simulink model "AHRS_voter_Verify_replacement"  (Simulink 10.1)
settings: Solver=FixedStepDiscrete  StartTime=0.0  StopTime=10.0  RelTol=1e-3
undefined symbols (not defined in the file or in its folder): sldvsubsys
libraries: simulink x2, sldvlib x1

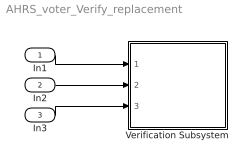
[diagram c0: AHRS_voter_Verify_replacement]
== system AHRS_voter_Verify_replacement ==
  In1 : Inport  OutDataTypeStr=Bus: AHRS_Bus
  In2 : Inport  Port=2  OutDataTypeStr=Bus: AHRS_Bus
  In3 : Inport  Port=3  OutDataTypeStr=Bus: AHRS_Bus
  Verification Subsystem : Subsystem  Tag=VerificationSubsystem  DisableCoverage=on  LoadFcn=sldvsubsys('check')  TreatAsAtomicUnit=on  SimViewingDevice=on
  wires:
  In1/1 -> Verification Subsystem/1(In1)
  In2/1 -> Verification Subsystem/2(In2)
  In3/1 -> Verification Subsystem/3(In3)

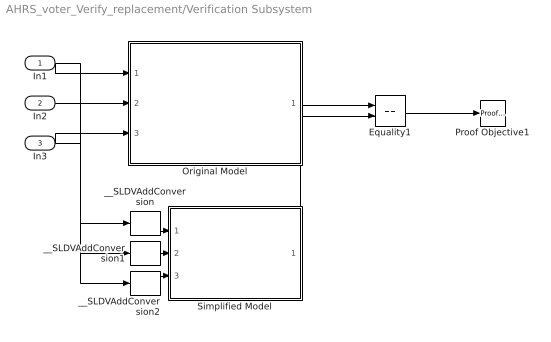
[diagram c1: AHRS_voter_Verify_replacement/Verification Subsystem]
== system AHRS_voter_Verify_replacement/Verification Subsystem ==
  In1 : Inport  OutDataTypeStr=Bus: AHRS_Bus
  In2 : Inport  Port=2  OutDataTypeStr=Bus: AHRS_Bus
  In3 : Inport  Port=3  OutDataTypeStr=Bus: AHRS_Bus
  Equality1 : RelationalOperator  Operator===  OutDataTypeStr=boolean  RndMeth=Simplest
  Original Model : Subsystem  TreatAsAtomicUnit=on
  Proof Objective1 : sldvlib/Objectives and Constraints/Proof Objective  enabled=on  customAVTBlockType=Proof Objective  intervals=true  dispValues=on  outEnabled=off  enableStopSim=off
  Simplified Model : Subsystem  TreatAsAtomicUnit=on
  __SLDVAddConversion : SignalConversion  ConversionOutput=Nonvirtual bus  OutDataTypeStr=Bus:AHRS_Bus  OverrideOpt=off
  __SLDVAddConversion1 : SignalConversion  ConversionOutput=Nonvirtual bus  OutDataTypeStr=Bus:AHRS_Bus  OverrideOpt=off
  __SLDVAddConversion2 : SignalConversion  ConversionOutput=Nonvirtual bus  OutDataTypeStr=Bus:AHRS_Bus  OverrideOpt=off
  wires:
  In1/1 -> Original Model/1(AHRS1), __SLDVAddConversion/1
  In2/1 -> Original Model/2(AHRS2), __SLDVAddConversion1/1
  In3/1 -> Original Model/3(AHRS3), __SLDVAddConversion2/1
  Original Model/1(voted_fb) -> Equality1/1
  Simplified Model/1(voted_fb) -> Equality1/2
  Equality1/1 -> Proof Objective1/1
  __SLDVAddConversion/1 -> Simplified Model/1(AHRS1)
  __SLDVAddConversion1/1 -> Simplified Model/2(AHRS2)
  __SLDVAddConversion2/1 -> Simplified Model/3(AHRS3)

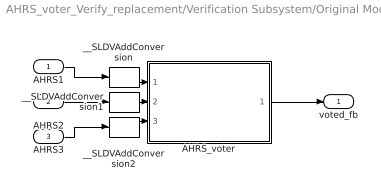
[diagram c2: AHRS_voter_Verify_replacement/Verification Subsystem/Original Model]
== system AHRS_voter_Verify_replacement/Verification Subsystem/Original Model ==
  AHRS1 : Inport  OutDataTypeStr=Bus: AHRS_Bus  SampleTime=[0.01,0]
  AHRS2 : Inport  Port=2  OutDataTypeStr=Bus: AHRS_Bus  SampleTime=[0.01,0]
  AHRS3 : Inport  Port=3  OutDataTypeStr=Bus: AHRS_Bus  SampleTime=[0.01,0]
  AHRS_voter : Subsystem  TreatAsAtomicUnit=on
  __SLDVAddConversion : SignalConversion  ConversionOutput=Nonvirtual bus  OutDataTypeStr=Bus:AHRS_Bus  OverrideOpt=off
  __SLDVAddConversion1 : SignalConversion  ConversionOutput=Nonvirtual bus  OutDataTypeStr=Bus:AHRS_Bus  OverrideOpt=off
  __SLDVAddConversion2 : SignalConversion  ConversionOutput=Nonvirtual bus  OutDataTypeStr=Bus:AHRS_Bus  OverrideOpt=off
  voted_fb : Outport  OutDataTypeStr=double  PortDimensions=5  SampleTime=[0.01,0]
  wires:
  AHRS_voter/1(voted_fb) -> voted_fb/1
  AHRS1/1 -> __SLDVAddConversion/1
  __SLDVAddConversion/1 -> AHRS_voter/1(AHRS1)
  AHRS2/1 -> __SLDVAddConversion1/1
  __SLDVAddConversion1/1 -> AHRS_voter/2(AHRS2)
  AHRS3/1 -> __SLDVAddConversion2/1
  __SLDVAddConversion2/1 -> AHRS_voter/3(AHRS3)

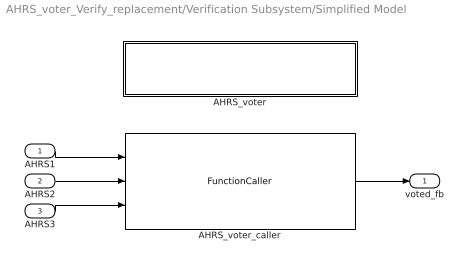
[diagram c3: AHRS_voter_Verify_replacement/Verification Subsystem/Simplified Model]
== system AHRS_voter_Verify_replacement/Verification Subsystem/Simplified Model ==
  AHRS1 : Inport  OutDataTypeStr=Bus: AHRS_Bus  SampleTime=[0.01,0]
  AHRS2 : Inport  Port=2  OutDataTypeStr=Bus: AHRS_Bus  SampleTime=[0.01,0]
  AHRS3 : Inport  Port=3  OutDataTypeStr=Bus: AHRS_Bus  SampleTime=[0.01,0]
  AHRS_voter : Subsystem  TreatAsAtomicUnit=on
  AHRS_voter_caller : FunctionCaller  FunctionPrototype=voted_fb = AHRS_voter(AHRS1,AHRS2,AHRS3)
  voted_fb : Outport  OutDataTypeStr=double  PortDimensions=5  SampleTime=[0.01,0]
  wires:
  AHRS_voter_caller/1 -> voted_fb/1
  AHRS3/1 -> AHRS_voter_caller/3
  AHRS2/1 -> AHRS_voter_caller/2
  AHRS1/1 -> AHRS_voter_caller/1

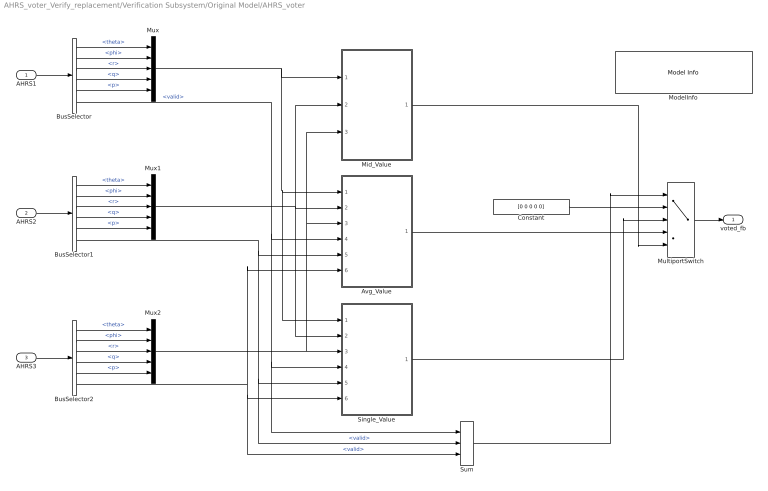
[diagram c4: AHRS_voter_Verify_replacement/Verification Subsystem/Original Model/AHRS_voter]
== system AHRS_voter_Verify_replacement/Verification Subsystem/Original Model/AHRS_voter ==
  AHRS1 : Inport  OutDataTypeStr=Bus: AHRS_Bus  PortDimensions=1  SampleTime=[0.01,0]
  AHRS2 : Inport  Port=2  OutDataTypeStr=Bus: AHRS_Bus  PortDimensions=1  SampleTime=[0.01,0]
  AHRS3 : Inport  Port=3  OutDataTypeStr=Bus: AHRS_Bus  PortDimensions=1  SampleTime=[0.01,0]
  Avg_Value : Subsystem  TreatAsAtomicUnit=on  RTWFcnName=Avg_Value
  BusSelector : BusSelector  OutputSignals=theta,phi,r,q,p,valid
  BusSelector1 : BusSelector  OutputSignals=theta,phi,r,q,p,valid
  BusSelector2 : BusSelector  OutputSignals=theta,phi,r,q,p,valid
  Constant : Constant  Value=[0 0 0 0 0]
  Mid_Value : Subsystem  TreatAsAtomicUnit=on  RTWFcnName=Mid_Value
  ModelInfo : simulink/Model-Wide Utilities/Model Info  Frame=on  DisplayStringWithTags=|  HorizontalTextAlignment=Center  LeftAlignmentValue=0.5
      | Model Name: %<ModelName>
      | Model Version: %<ModelVersion>
      | Last Modified: %<LastModificationDate>
      | 
      | Copyright 2016 The MathWorks, Inc.
  MultiportSwitch : MultiPortSwitch  DataPortOrder=Zero-based contiguous  Inputs=4  DiagnosticForDefault=None  zeroidx=on
  Mux : Mux  Inputs=5
  Mux1 : Mux  Inputs=5
  Mux2 : Mux  Inputs=5
  Single_Value : Subsystem  TreatAsAtomicUnit=on  RTWFcnName=Single_Value
  Sum : Sum  Inputs=+++  OutDataTypeStr=uint32
  voted_fb : Outport  OutDataTypeStr=double  PortDimensions=5  SampleTime=[0.01,0]  VectorParamsAs1DForOutWhenUnconnected=off
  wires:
  BusSelector2/6 -> Single_Value/6(AHRS3_Valid), Sum/3, Avg_Value/6(AHRS3_Valid)  "<valid>"
  BusSelector2/5 -> Mux2/5  "<p>"
  BusSelector2/4 -> Mux2/4  "<q>"
  BusSelector2/3 -> Mux2/3  "<r>"
  BusSelector2/2 -> Mux2/2  "<phi>"
  BusSelector2/1 -> Mux2/1  "<theta>"
  AHRS3/1 -> BusSelector2/1
  Mux2/1 -> Mid_Value/3(AHRS3), Avg_Value/3(AHRS3), Single_Value/3(AHRS3)
  BusSelector1/6 -> Avg_Value/5(AHRS2_Valid), Sum/2, Single_Value/5(AHRS2_Valid)  "<valid>"
  Mux1/1 -> Single_Value/2(AHRS2), Mid_Value/2(AHRS2), Avg_Value/2(AHRS2)
  AHRS2/1 -> BusSelector1/1
  BusSelector1/1 -> Mux1/1  "<theta>"
  BusSelector1/2 -> Mux1/2  "<phi>"
  BusSelector1/3 -> Mux1/3  "<r>"
  BusSelector1/4 -> Mux1/4  "<q>"
  BusSelector1/5 -> Mux1/5  "<p>"
  Mux/1 -> Single_Value/1(AHRS1), Avg_Value/1(AHRS1), Mid_Value/1(AHRS1)
  BusSelector/5 -> Mux/5  "<p>"
  BusSelector/4 -> Mux/4  "<q>"
  BusSelector/3 -> Mux/3  "<r>"
  BusSelector/2 -> Mux/2  "<phi>"
  BusSelector/1 -> Mux/1  "<theta>"
  BusSelector/6 -> Single_Value/4(AHRS1_Valid), Sum/1, Avg_Value/4(AHRS1_Valid)  "<valid>"
  AHRS1/1 -> BusSelector/1
  Constant/1 -> MultiportSwitch/2
  Single_Value/1(Single_Value) -> MultiportSwitch/3
  Avg_Value/1(Avg_Value) -> MultiportSwitch/4
  Mid_Value/1(Mid_Value) -> MultiportSwitch/5
  Sum/1 -> MultiportSwitch/1
  MultiportSwitch/1 -> voted_fb/1

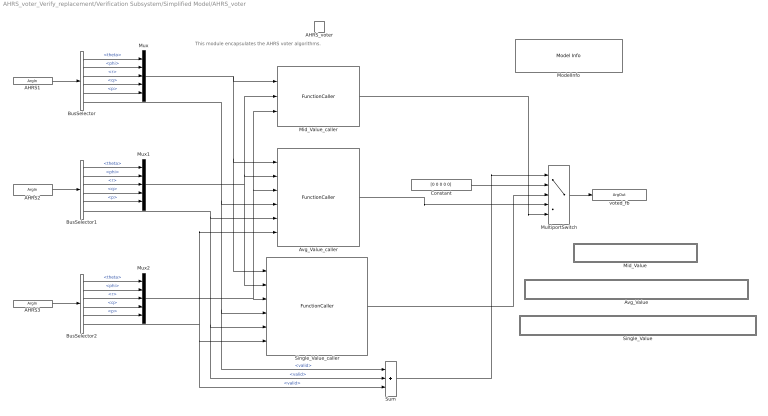
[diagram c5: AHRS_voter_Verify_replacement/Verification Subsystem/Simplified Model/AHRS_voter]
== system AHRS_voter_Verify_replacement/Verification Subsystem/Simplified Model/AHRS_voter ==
  note: This module encapsulates the AHRS voter algorithms.
  AHRS_voter : TriggerPort  TriggerType=function-call  IsSimulinkFunction=on  FunctionName=AHRS_voter  FunctionVisibility=scoped  VariantControl=Variant  PortDimensions=1
  Avg_Value : Subsystem  TreatAsAtomicUnit=on  RTWFcnName=Avg_Value
  Avg_Value_caller : FunctionCaller  FunctionPrototype=Avg_Value = Avg_Value(AHRS1,AHRS2,AHRS3,AHRS1_Valid,AHRS2_Valid,AHRS3_Valid)
  BusSelector : BusSelector  OutputSignals=theta,phi,r,q,p,valid
  BusSelector1 : BusSelector  OutputSignals=theta,phi,r,q,p,valid
  BusSelector2 : BusSelector  OutputSignals=theta,phi,r,q,p,valid
  Constant : Constant  Value=[0 0 0 0 0]
  Mid_Value : Subsystem  TreatAsAtomicUnit=on  RTWFcnName=Mid_Value
  Mid_Value_caller : FunctionCaller  FunctionPrototype=Mid_Value = Mid_Value(AHRS1,AHRS2,AHRS3)
  ModelInfo : simulink/Model-Wide Utilities/Model Info  Frame=on  DisplayStringWithTags=|  HorizontalTextAlignment=Center  LeftAlignmentValue=0.5
      | Model Name: %<ModelName>
      | Model Version: %<ModelVersion>
      | Last Modified: %<LastModificationDate>
      | 
      | Copyright 2016 The MathWorks, Inc.
  MultiportSwitch : MultiPortSwitch  DataPortOrder=Zero-based contiguous  Inputs=4  DiagnosticForDefault=None  zeroidx=on
  Mux : Mux  Inputs=5
  Mux1 : Mux  Inputs=5
  Mux2 : Mux  Inputs=5
  Single_Value : Subsystem  TreatAsAtomicUnit=on  RTWFcnName=Single_Value
  Single_Value_caller : FunctionCaller  FunctionPrototype=Single_Value = Single_Value(AHRS1,AHRS2,AHRS3,AHRS1_Valid,AHRS2_Valid,AHRS3_Valid)
  Sum : Sum  Inputs=+++  OutDataTypeStr=uint32
  AHRS1 : ArgIn  OutDataTypeStr=Bus: AHRS_Bus  ArgumentName=AHRS1
  AHRS2 : ArgIn  Port=2  OutDataTypeStr=Bus: AHRS_Bus  ArgumentName=AHRS2
  AHRS3 : ArgIn  Port=3  OutDataTypeStr=Bus: AHRS_Bus  ArgumentName=AHRS3
  voted_fb : ArgOut  PortDimensions=5  ArgumentName=voted_fb
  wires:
  BusSelector2/5 -> Mux2/5  "<p>"
  Mux2/1 -> Avg_Value_caller/3, Mid_Value_caller/3, Single_Value_caller/3
  BusSelector/4 -> Mux/4  "<q>"
  BusSelector2/1 -> Mux2/1  "<theta>"
  BusSelector/2 -> Mux/2  "<phi>"
  BusSelector2/2 -> Mux2/2  "<phi>"
  BusSelector2/3 -> Mux2/3  "<r>"
  BusSelector1/2 -> Mux1/2  "<phi>"
  Sum/1 -> MultiportSwitch/1
  BusSelector1/4 -> Mux1/4  "<q>"
  Constant/1 -> MultiportSwitch/2
  BusSelector2/4 -> Mux2/4  "<q>"
  BusSelector2/6 -> Sum/3, Single_Value_caller/6, Avg_Value_caller/6  "<valid>"
  BusSelector/6 -> Sum/1, Single_Value_caller/4, Avg_Value_caller/4  "<valid>"
  BusSelector1/3 -> Mux1/3  "<r>"
  BusSelector/1 -> Mux/1  "<theta>"
  Mux/1 -> Mid_Value_caller/1, Single_Value_caller/1, Avg_Value_caller/1
  BusSelector/3 -> Mux/3  "<r>"
  Single_Value_caller/1 -> MultiportSwitch/3
  BusSelector1/1 -> Mux1/1  "<theta>"
  BusSelector1/5 -> Mux1/5  "<p>"
  Mux1/1 -> Single_Value_caller/2, Avg_Value_caller/2, Mid_Value_caller/2
  BusSelector/5 -> Mux/5  "<p>"
  MultiportSwitch/1 -> voted_fb/1
  Mid_Value_caller/1 -> MultiportSwitch/5
  Avg_Value_caller/1 -> MultiportSwitch/4
  BusSelector1/6 -> Sum/2, Single_Value_caller/5, Avg_Value_caller/5  "<valid>"
  AHRS1/1 -> BusSelector/1
  AHRS2/1 -> BusSelector1/1
  AHRS3/1 -> BusSelector2/1

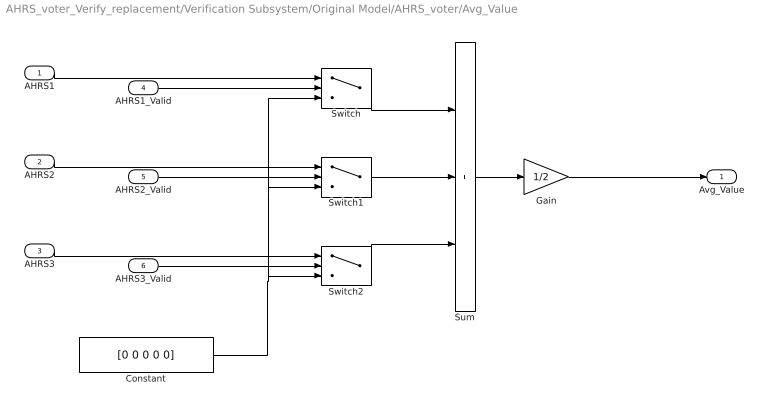
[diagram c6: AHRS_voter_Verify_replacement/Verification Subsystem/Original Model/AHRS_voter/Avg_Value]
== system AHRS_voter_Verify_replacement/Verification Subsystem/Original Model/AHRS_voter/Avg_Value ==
  AHRS1 : Inport
  AHRS2 : Inport  Port=2
  AHRS3 : Inport  Port=3
  AHRS1_Valid : Inport  Port=4  OutDataTypeStr=boolean  PortDimensions=1
  AHRS2_Valid : Inport  Port=5  OutDataTypeStr=boolean  PortDimensions=1
  AHRS3_Valid : Inport  Port=6  OutDataTypeStr=boolean  PortDimensions=1
  Constant : Constant  Value=[0 0 0 0 0]
  Gain : Gain  Gain=1/2
  Sum : Sum  Inputs=+++
  Switch : Switch  Criteria=u2 ~= 0
  Switch1 : Switch  Criteria=u2 ~= 0
  Switch2 : Switch  Criteria=u2 ~= 0
  Avg_Value : Outport  VectorParamsAs1DForOutWhenUnconnected=off
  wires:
  Gain/1 -> Avg_Value/1
  Sum/1 -> Gain/1
  AHRS1_Valid/1 -> Switch/2
  AHRS1/1 -> Switch/1
  Switch/1 -> Sum/1
  Switch1/1 -> Sum/2
  Switch2/1 -> Sum/3
  AHRS2_Valid/1 -> Switch1/2
  AHRS3_Valid/1 -> Switch2/2
  AHRS2/1 -> Switch1/1
  AHRS3/1 -> Switch2/1
  Constant/1 -> Switch/3, Switch1/3, Switch2/3

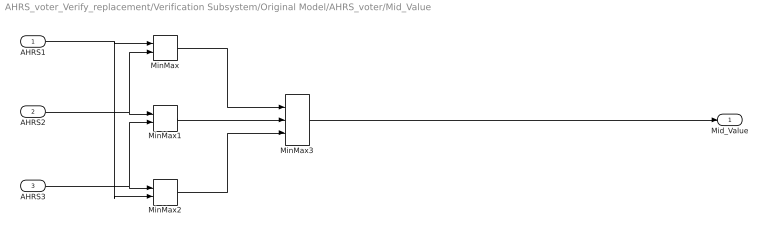
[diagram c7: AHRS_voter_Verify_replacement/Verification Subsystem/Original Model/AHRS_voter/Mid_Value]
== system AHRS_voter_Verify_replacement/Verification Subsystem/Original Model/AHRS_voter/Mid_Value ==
  AHRS1 : Inport
  AHRS2 : Inport  Port=2
  AHRS3 : Inport  Port=3
  MinMax : MinMax  Inputs=2
  MinMax1 : MinMax  Inputs=2
  MinMax2 : MinMax  Inputs=2
  MinMax3 : MinMax  Function=max  Inputs=3
  Mid_Value : Outport  VectorParamsAs1DForOutWhenUnconnected=off
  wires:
  AHRS1/1 -> MinMax2/2, MinMax/1
  AHRS3/1 -> MinMax1/2, MinMax2/1
  AHRS2/1 -> MinMax/2, MinMax1/1
  MinMax1/1 -> MinMax3/2
  MinMax/1 -> MinMax3/1
  MinMax2/1 -> MinMax3/3
  MinMax3/1 -> Mid_Value/1

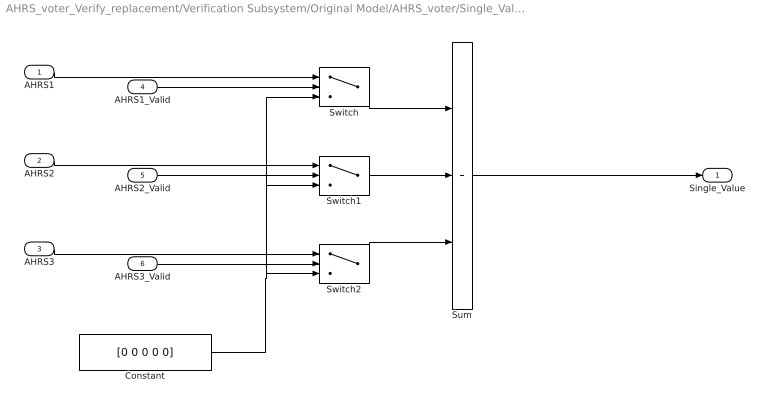
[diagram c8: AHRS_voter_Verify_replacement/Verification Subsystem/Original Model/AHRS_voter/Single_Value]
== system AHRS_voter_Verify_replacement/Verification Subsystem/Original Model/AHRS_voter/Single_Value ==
  AHRS1 : Inport
  AHRS2 : Inport  Port=2
  AHRS3 : Inport  Port=3
  AHRS1_Valid : Inport  Port=4  OutDataTypeStr=boolean  PortDimensions=1
  AHRS2_Valid : Inport  Port=5  OutDataTypeStr=boolean  PortDimensions=1
  AHRS3_Valid : Inport  Port=6  OutDataTypeStr=boolean  PortDimensions=1
  Constant : Constant  Value=[0 0 0 0 0]
  Sum : Sum  Inputs=+++
  Switch : Switch  Criteria=u2 ~= 0
  Switch1 : Switch  Criteria=u2 ~= 0
  Switch2 : Switch  Criteria=u2 ~= 0
  Single_Value : Outport  VectorParamsAs1DForOutWhenUnconnected=off
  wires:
  Constant/1 -> Switch2/3, Switch1/3, Switch/3
  AHRS3/1 -> Switch2/1
  AHRS2/1 -> Switch1/1
  AHRS3_Valid/1 -> Switch2/2
  AHRS2_Valid/1 -> Switch1/2
  Switch2/1 -> Sum/3
  Switch1/1 -> Sum/2
  Switch/1 -> Sum/1
  AHRS1/1 -> Switch/1
  AHRS1_Valid/1 -> Switch/2
  Sum/1 -> Single_Value/1

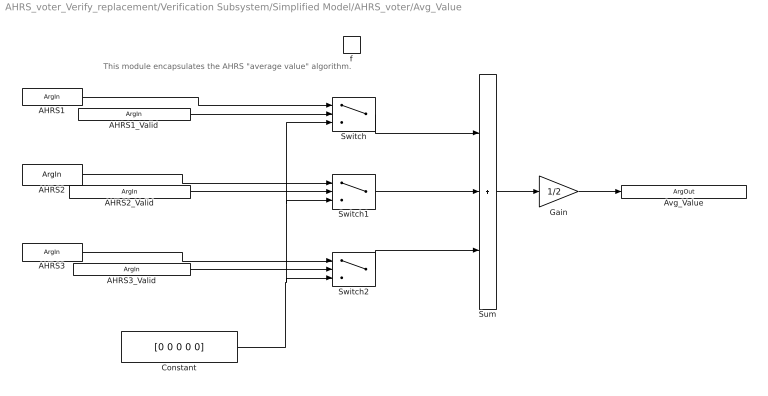
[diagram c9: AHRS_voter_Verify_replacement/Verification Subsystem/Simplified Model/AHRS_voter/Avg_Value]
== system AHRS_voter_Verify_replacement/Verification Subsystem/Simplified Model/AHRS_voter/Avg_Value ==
  note: This module encapsulates the AHRS "average value" algorithm.
  f : TriggerPort  TriggerType=function-call  IsSimulinkFunction=on  FunctionName=Avg_Value  FunctionVisibility=scoped  VariantControl=Variant  PortDimensions=1
  Constant : Constant  Value=[0 0 0 0 0]
  Gain : Gain  Gain=1/2
  Sum : Sum  Inputs=+++
  Switch : Switch  Criteria=u2 ~= 0
  Switch1 : Switch  Criteria=u2 ~= 0
  Switch2 : Switch  Criteria=u2 ~= 0
  AHRS1 : ArgIn  PortDimensions=5  ArgumentName=AHRS1
  AHRS2 : ArgIn  Port=2  PortDimensions=5  ArgumentName=AHRS2
  AHRS3 : ArgIn  Port=3  PortDimensions=5  ArgumentName=AHRS3
  AHRS1_Valid : ArgIn  Port=4  OutDataTypeStr=boolean  ArgumentName=AHRS1_Valid
  AHRS2_Valid : ArgIn  Port=5  OutDataTypeStr=boolean  ArgumentName=AHRS2_Valid
  AHRS3_Valid : ArgIn  Port=6  OutDataTypeStr=boolean  ArgumentName=AHRS3_Valid
  Avg_Value : ArgOut  PortDimensions=5  ArgumentName=Avg_Value
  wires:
  Gain/1 -> Avg_Value/1
  Sum/1 -> Gain/1
  AHRS1_Valid/1 -> Switch/2
  AHRS1/1 -> Switch/1
  Switch/1 -> Sum/1
  Switch1/1 -> Sum/2
  Switch2/1 -> Sum/3
  AHRS2_Valid/1 -> Switch1/2
  AHRS3_Valid/1 -> Switch2/2
  AHRS2/1 -> Switch1/1
  AHRS3/1 -> Switch2/1
  Constant/1 -> Switch/3, Switch1/3, Switch2/3

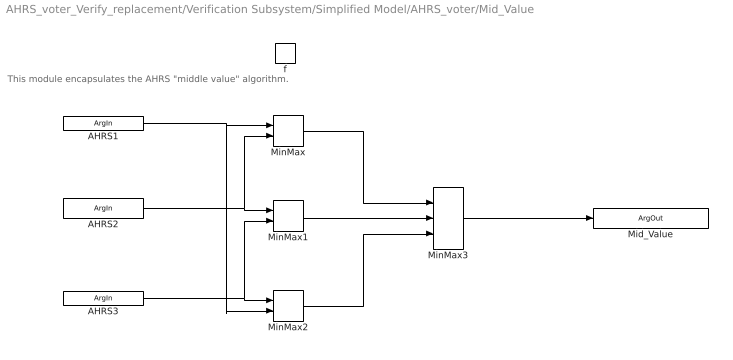
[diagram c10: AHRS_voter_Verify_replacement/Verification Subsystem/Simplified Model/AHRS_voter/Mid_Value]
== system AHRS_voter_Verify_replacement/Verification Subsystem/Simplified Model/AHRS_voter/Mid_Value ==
  note: This module encapsulates the AHRS "middle value" algorithm.
  f : TriggerPort  TriggerType=function-call  IsSimulinkFunction=on  FunctionName=Mid_Value  FunctionVisibility=scoped  VariantControl=Variant  PortDimensions=1
  MinMax : MinMax  Inputs=2
  MinMax1 : MinMax  Inputs=2
  MinMax2 : MinMax  Inputs=2
  MinMax3 : MinMax  Function=max  Inputs=3
  AHRS1 : ArgIn  PortDimensions=5  ArgumentName=AHRS1
  AHRS2 : ArgIn  Port=2  PortDimensions=5  ArgumentName=AHRS2
  AHRS3 : ArgIn  Port=3  PortDimensions=5  ArgumentName=AHRS3
  Mid_Value : ArgOut  PortDimensions=5  ArgumentName=Mid_Value
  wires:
  AHRS1/1 -> MinMax2/2, MinMax/1
  AHRS3/1 -> MinMax1/2, MinMax2/1
  AHRS2/1 -> MinMax/2, MinMax1/1
  MinMax1/1 -> MinMax3/2
  MinMax/1 -> MinMax3/1
  MinMax2/1 -> MinMax3/3
  MinMax3/1 -> Mid_Value/1

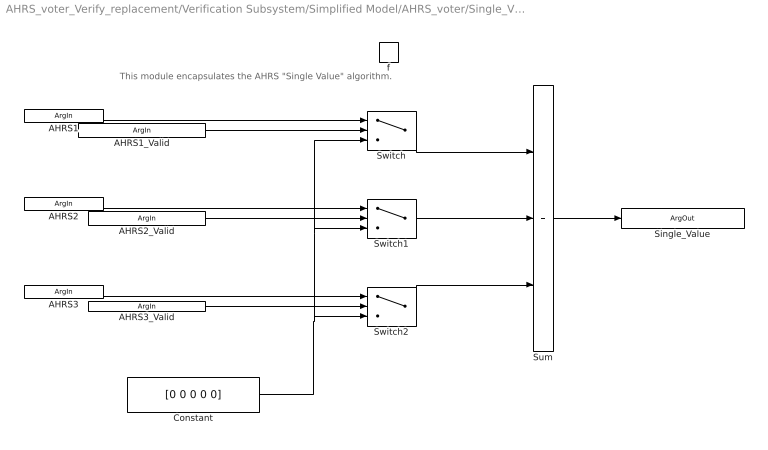
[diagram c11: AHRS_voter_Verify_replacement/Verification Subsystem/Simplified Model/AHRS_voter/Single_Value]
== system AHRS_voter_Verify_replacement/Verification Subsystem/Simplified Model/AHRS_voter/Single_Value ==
  note: This module encapsulates the AHRS "Single Value" algorithm.
  f : TriggerPort  TriggerType=function-call  IsSimulinkFunction=on  FunctionName=Single_Value  FunctionVisibility=scoped  VariantControl=Variant  PortDimensions=1
  Constant : Constant  Value=[0 0 0 0 0]
  Sum : Sum  Inputs=+++
  Switch : Switch  Criteria=u2 ~= 0
  Switch1 : Switch  Criteria=u2 ~= 0
  Switch2 : Switch  Criteria=u2 ~= 0
  AHRS1 : ArgIn  PortDimensions=5  ArgumentName=AHRS1
  AHRS2 : ArgIn  Port=2  PortDimensions=5  ArgumentName=AHRS2
  AHRS3 : ArgIn  Port=3  PortDimensions=5  ArgumentName=AHRS3
  AHRS1_Valid : ArgIn  Port=4  OutDataTypeStr=boolean  ArgumentName=AHRS1_Valid
  AHRS2_Valid : ArgIn  Port=5  OutDataTypeStr=boolean  ArgumentName=AHRS2_Valid
  AHRS3_Valid : ArgIn  Port=6  OutDataTypeStr=boolean  ArgumentName=AHRS3_Valid
  Single_Value : ArgOut  PortDimensions=5  ArgumentName=Single_Value
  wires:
  Constant/1 -> Switch2/3, Switch1/3, Switch/3
  AHRS3/1 -> Switch2/1
  AHRS2/1 -> Switch1/1
  AHRS3_Valid/1 -> Switch2/2
  AHRS2_Valid/1 -> Switch1/2
  Switch2/1 -> Sum/3
  Switch1/1 -> Sum/2
  Switch/1 -> Sum/1
  AHRS1/1 -> Switch/1
  AHRS1_Valid/1 -> Switch/2
  Sum/1 -> Single_Value/1
